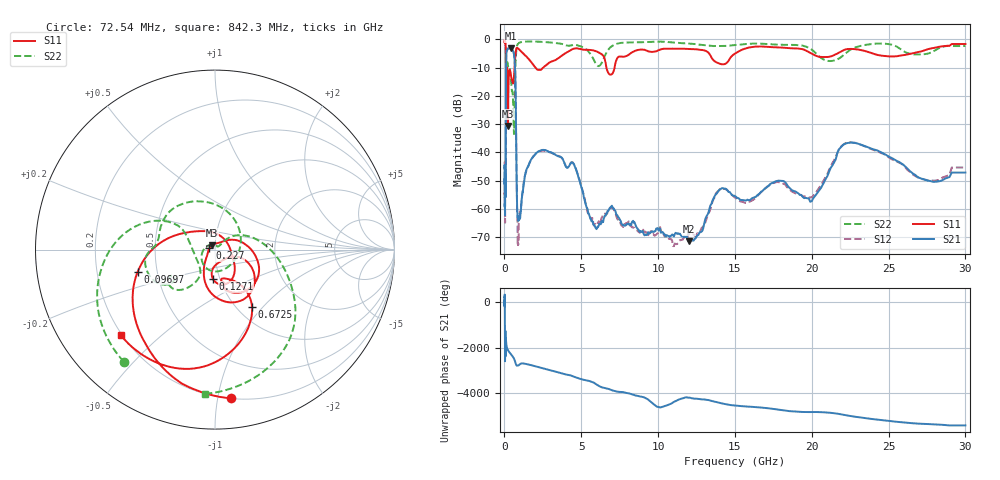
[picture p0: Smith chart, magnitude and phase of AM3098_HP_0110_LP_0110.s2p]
! Date/Time: Thu, Feb 28, 2019 8:37 AM
! Network Analyzer: Agilent Technologies E8364B Rev: A.07.50.67
! Sweep from 0.010 to 30.000 GHz, 1601 Points, Sweep Type: LOG
! Power Supply: 5.023 V, 0.002 A
# Hz S DB R 50
!freq MagS11 AngS11 MagS21 AngS21 MagS12 AngS12 MagS22 AngS22
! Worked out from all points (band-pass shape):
!   1601 points, 10 MHz to 30 GHz, reference 50 ohm
!   highest |S21| = -3.11 dB at 413.9 MHz (marker M1); lowest = -71.4 dB at 12.01 GHz (marker M2)
!   |S21| within 3 dB of the highest: 117.2 MHz to 640.9 MHz (523.7 MHz wide, 138 % of centre)
!   lowest |S11| = -30.7 dB at 231.6 MHz (marker M3), VSWR 1.06, Z = 48.3 + j2.37 ohm
!   |S11| at or under -10 dB: 176.2 MHz to 655.8 MHz (479.7 MHz wide, 115 % of centre); 2.028 GHz to 2.519 GHz (491.4 MHz wide, 21.6 % of centre); 6.64 GHz to 7.164 GHz (524.8 MHz wide, 7.6 % of centre)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
!   |S22| runs from -33.5 to -0.5 dB; largest |S21 - S12| = 0.011
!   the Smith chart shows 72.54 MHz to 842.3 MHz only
!   S11 on the Smith chart (normalised r, x): 72.54 MHz: 0.20, -1.09; 96.97 MHz: 0.39, -0.12; 127.1 MHz: 0.93, -0.31; 227 MHz: 0.94, +0.02; 672.5 MHz: 1.17, -0.87; 842.3 MHz: 0.20, -0.37
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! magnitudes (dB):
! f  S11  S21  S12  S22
! 10 MHz  -0.4  -45.7  -43.2  -0.5
! 38.04 MHz  -0.5  -61.0  -62.6  -0.8
! 72.54 MHz  -1.6  -55.9  -54.4  -1.9
! 84.71 MHz  -2.7  -50.4  -50.5  -2.9
! 96.97 MHz  -7.0  -24.7  -24.6  -8.0
! 127.1 MHz  -15.8  -5.0  -5.0  -10.0
! 144.7 MHz  -18.4  -4.0  -3.9  -11.1
! 184 MHz  -10.6  -3.7  -3.7  -8.0
! 227 MHz  -29.9  -3.3  -3.2  -9.4
! 231.6 MHz  -30.7  -3.2  -3.2  -9.5
! 413.9 MHz  -12.6  -3.1  -3.1  -13.5
! 550.5 MHz  -15.6  -3.9  -3.9  -20.5
! 620.7 MHz  -13.2  -5.3  -5.2  -33.4
! 672.5 MHz  -8.4  -8.3  -8.3  -19.3
! 842.3 MHz  -3.0  -62.1  -63.5  -1.9
! 2.084 GHz  -10.4  -40.2  -40.1  -0.8
! 7.926 GHz  -5.9  -65.7  -65.0  -1.1
! 12.01 GHz  -3.4  -71.4  -68.9  -1.4
! 14.09 GHz  -8.7  -52.9  -52.9  -2.3
! 20 GHz  -5.0  -57.2  -55.9  -3.6
! 22.56 GHz  -3.3  -36.5  -36.4  -3.5
! 30 GHz  -1.6  -47.1  -45.3  -2.3
